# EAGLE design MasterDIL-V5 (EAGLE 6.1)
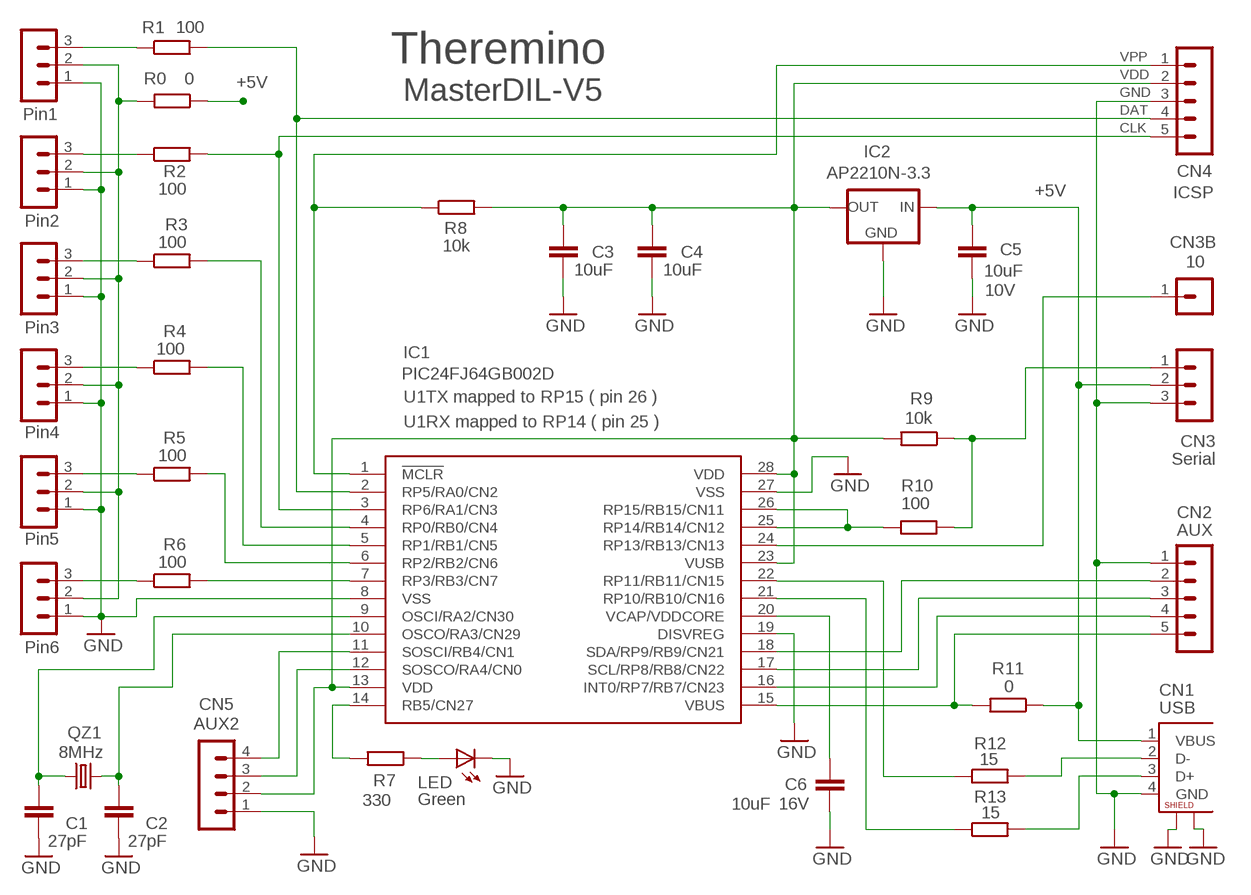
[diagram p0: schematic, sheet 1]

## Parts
C1  27pF  C-EUC0603  [C0603]
C2  27pF  C-EUC0603  [C0603]
C3  10uF  C-EUC0805  [C0805]
C4  10uF  C-EUC0805  [C0805]
C5  10uF  C-EUC0805  [C0805]
C6  10uF  C-EUC0805  [C0805]
CN1  USB  USB-BL  [USB-B-LARGE]
CN2  AUX  MA05-1  [MA05-1]
CN3  Serial  MA03-1N  [MA03-1]
CN3B  10  MA01-1  [MA01-1]
CN4  ICSP  MA05-1  [MA05-1]
CN5  AUX2  MA04-1  [MA04-1]
IC1  PIC24FJ64GB002D  [DIL28-3]
IC2  AP2210N-3.3  MCP1700SOT23L  [SOT23_L]
LED  Green  LEDLED3MM  [LED3MM]
QZ1  8MHz  CRYSTALHC49U70  [HC49U70]
R0  0  R-EU_R1206_L  [R1206_L]
R1  100  R-EU_R1206_L  [R1206_L]
R2  100  R-EU_R0805  [R0805]
R3  100  R-EU_R0805  [R0805]
R4  100  R-EU_R0805  [R0805]
R5  100  R-EU_R0805  [R0805]
R6  100  R-EU_R0805  [R0805]
R7  330  R-EU_R0805  [R0805]
R8  10k  R-EU_R0805  [R0805]
R9  10k  R-EU_R1206_L  [R1206_L]
R10  100  R-EU_R0805  [R0805]
R11  0  R-EU_R2512W  [R2512W]
R12  15  R-EU_R1206_L  [R1206_L]
R13  15  R-EU_R1206_L  [R1206_L]
SV1  Pin1  MA03-1L1  [MA03-1_L1]
SV2  Pin2  MA03-1L1  [MA03-1_L1]
SV3  Pin3  MA03-1L1  [MA03-1_L1]
SV4  Pin4  MA03-1L1  [MA03-1_L1]
SV5  Pin5  MA03-1L1  [MA03-1_L1]
SV6  Pin6  MA03-1L1  [MA03-1_L1]

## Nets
+5_PINS: R0.2 SV1.2 SV2.2 SV3.2 SV4.2 SV5.2 SV6.2
+5V: C5.1 CN1.1(VBUS) CN3.2 IC2.3(IN) R0.1 R11.1
GND: C1.2 C2.1 C3.2 C4.2 C5.2 C6.2 CN1.4(GND) CN1.G1 CN1.G2 CN2.1 CN3.3 CN4.3 CN5.1 IC1.8(VSS) IC1.19(DISVREG) IC1.27(VSS) IC2.1(GND) LED.K(C) SV1.1 SV2.1 SV3.1 SV4.1 SV5.1 SV6.1
N$1: CN4.1 IC1.1(!MCLR) R8.1
N$2: CN4.4 IC1.2(RP5/RA0/CN2) R1.2
N$3: IC1.21(RP10/RB10/CN16) R13.1
N$4: CN1.2(D-) R12.2
N$5: R1.1 SV1.3
N$6: CN4.5 IC1.3(RP6/RA1/CN3) R2.2
N$7: IC1.22(RP11/RB11/CN15) R12.1
N$8: LED.A R7.1
N$9: CN2.4 IC1.16(INT0/RP7/RB7/CN23)
N$10: CN5.3 IC1.12(SOSCO/RA4/CN0)
N$11: IC1.25(RP14/RB14/CN12) IC1.26(RP15/RB15/CN11) R10.1
N$12: CN2.3 IC1.17(SCL/RP8/RB8/CN22)
N$13: CN1.3(D+) R13.2
N$14: CN2.2 IC1.18(SDA/RP9/RB9/CN21)
N$15: CN3.1 R9.1 R10.2
N$16: C2.2 IC1.10(OSCO/RA3/CN29) QZ1.2
N$17: C1.1 IC1.9(OSCI/RA2/CN30) QZ1.1
N$18: CN3B.1 IC1.24(RP13/RB13/CN13)
N$19: IC1.7(RP3/RB3/CN7) R6.2
N$20: IC1.6(RP2/RB2/CN6) R5.2
N$21: IC1.5(RP1/RB1/CN5) R4.2
N$22: IC1.4(RP0/RB0/CN4) R3.2
N$23: R2.1 SV2.3
N$24: CN5.4 IC1.11(SOSCI/RB4/CN1)
N$25: R3.1 SV3.3
N$26: R4.1 SV4.3
N$27: R5.1 SV5.3
N$28: IC1.14(RB5/CN27) R7.2
N$29: R6.1 SV6.3
VBUS: CN2.5 IC1.15(VBUS) R11.2
VCAP/VDDCORE: C6.1 IC1.20(VCAP/VDDCORE)
VDD: C3.1 C4.1 CN4.2 CN5.2 IC1.13(VDD) IC1.23(VUSB) IC1.28(VDD) IC2.2(OUT) R8.2 R9.2

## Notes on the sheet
- Theremino
- MasterDIL-V5
- U1TX mapped to RP15 ( pin 26 )
- U1RX mapped to RP14 ( pin 25 )

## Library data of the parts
C1-C4 = 00-LIVIO:C-EU: CAPACITOR, European symbol
C5 = 00-LIVIO:C-EU: CAPACITOR, European symbol; VOLTAGE: 10V
C6 = 00-LIVIO:C-EU: CAPACITOR, European symbol; ESR: X5R; VOLTAGE: 16V
CN1 = 00-LIVIO:USB-B: USB Type-B Connector
CN2 = 03-con-lstb-M:MA05-1: PIN HEADER
CN3 SV1-SV6 = 03-con-lstb-M:MA03-1: PIN HEADER
CN3B = 03-con-lstb-M:MA01-1: PIN HEADER
CN4 = 03-con-lstb-M:MA05-1: PIN HEADER; CLK: CLK; DAT: DAT; GND: GND; VDD: VDD; VPP: VPP
CN5 = 03-con-lstb-M:MA04-1: PIN HEADER
IC1 = 00-LIVIO:PIC24FJ64GB002: PIC24FJ64GA002 edit this description Auto generated by make-symbol-device-package-bsdl.ulp Rev. 25 Source: PIC24FJ64GA002.bsd
IC2 = 00-LIVIO:MCP1700: Linear regulator Quescient courrent 1.8uA Input 2.3v to 6v Output 1.2v 1.8v 2.5v 3.0v 3.3v 5.0v
LED = 00-LIVIO:LED: LEDS
QZ1 = 00-LIVIO:CRYSTAL: CRYSTAL
R0 R1-R13 = 00-LIVIO:R-EU_: RESISTOR, European symbol

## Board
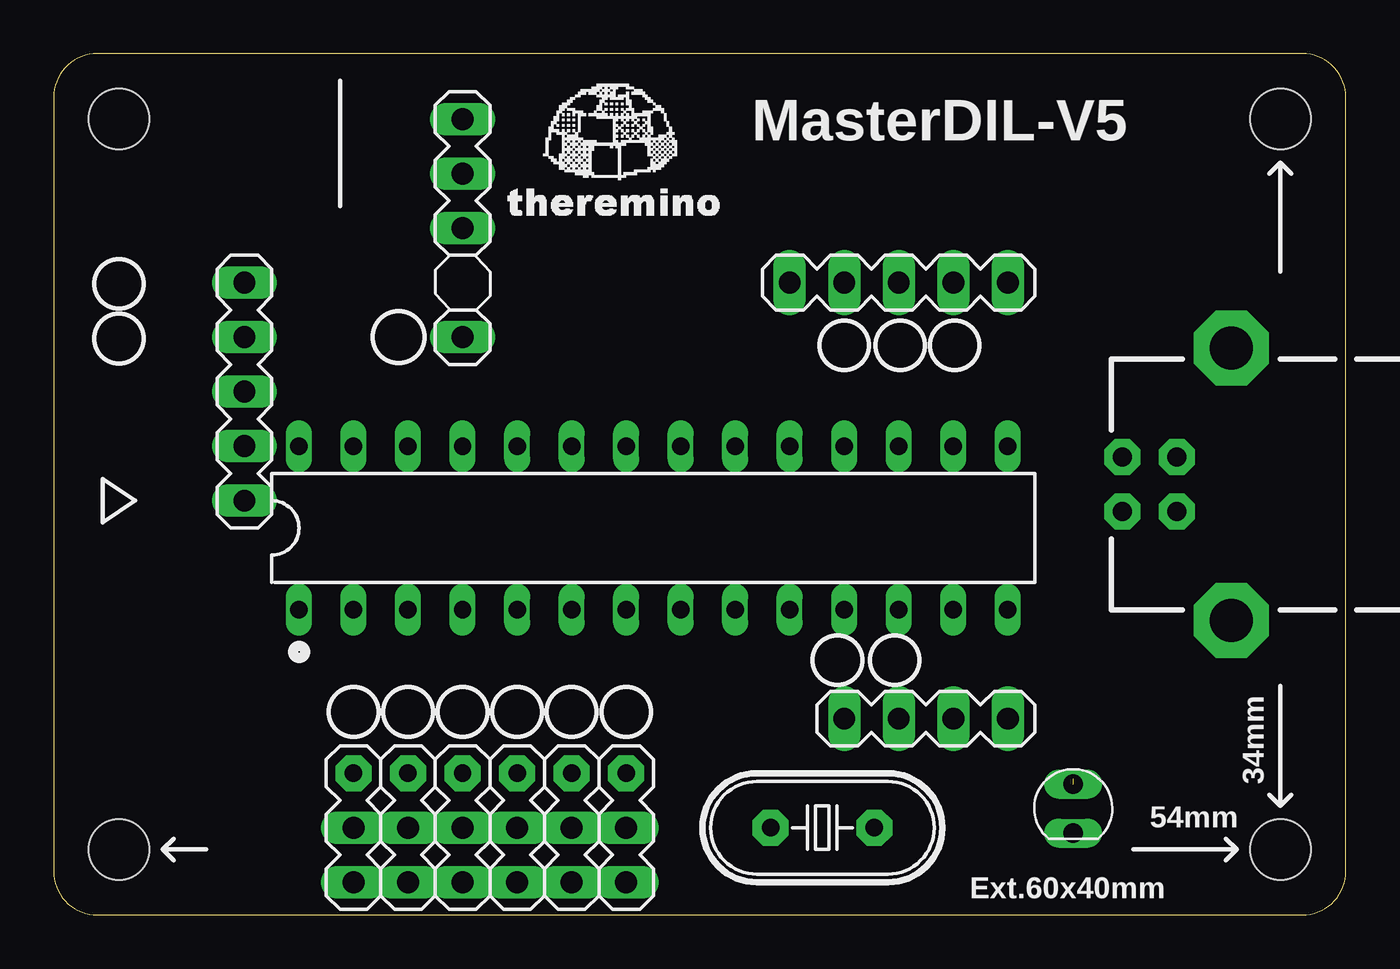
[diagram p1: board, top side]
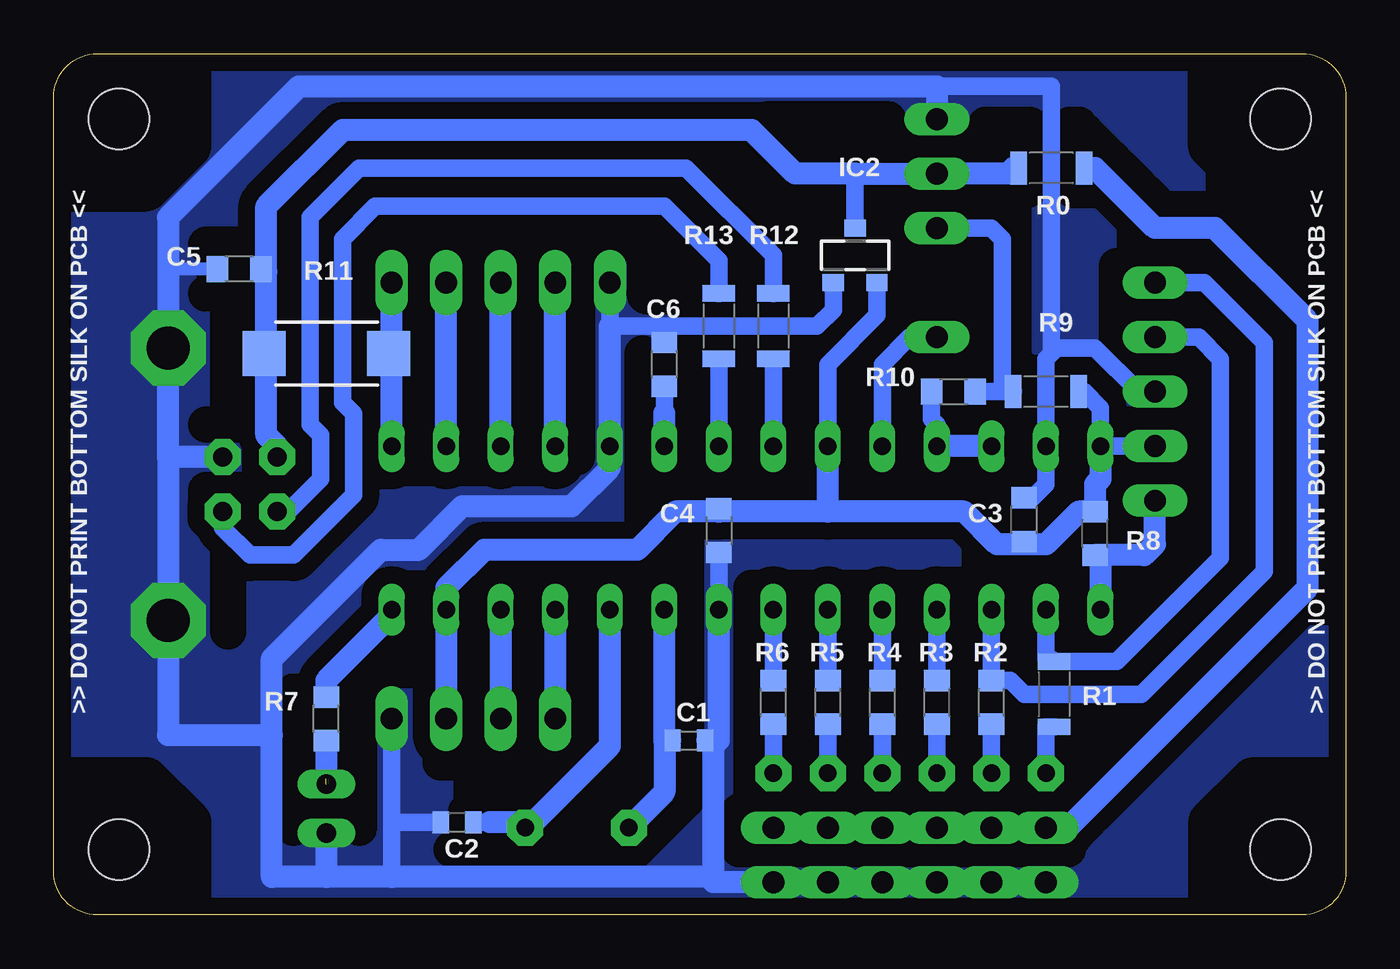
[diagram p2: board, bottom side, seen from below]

Size 60.2 x 40.13 mm. Coordinates in mm from the lower left corner, seen from the top.
Outline: 2.03,0 58.17,0 arc90 60.2,2.03 60.2,38.1 arc90 58.17,40.13 2.03,40.13 arc90 0,38.1 0,2.03 arc90 2.03,0
Copper layers (1*16): Top 0.035mm / dielectric 1.5mm / Bottom 0.035mm
Design rules: minimum track width 10mil, minimum drill 24mil, track to track 24mil, track to pad 24mil, pad to pad 24mil, via to via 24mil, smd to smd 24mil, copper to edge 24mil, drill to drill 8mil, minimum pad ring 5mil, minimum via ring 8mil, stop-mask expansion 4mil, vias tented up to drill 0mil, thermal gap 36mil
Holes 2.8 mm at 57.15,37.08 57.15,3.05 3.05,37.08 3.05,3.05
bRestrict: 67 lines

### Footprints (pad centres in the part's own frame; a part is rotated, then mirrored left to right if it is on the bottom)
C0603 = smd 0.762 x 1.016: 1 -0.762,0; 2 0.762,0
C0805 = smd 1 x 1.2: 1 -1.016,0; 2 1.016,0
USB-B-LARGE = drill 0.9 pad 1.676 octagon: 1 1.27,5.08; 2 -1.27,5.08; 3 -1.27,2.54; 4 1.27,2.54 | drill 2 pad 3.5 octagon: G1 -6.35,0; G2 6.35,0
MA05-1 = drill 1.016 long: 1 -5.08,0; 2 -2.54,0; 3 0,0; 4 2.54,0; 5 5.08,0
MA03-1 = drill 1.016 long: 1 -2.54,0; 2 0,0; 3 2.54,0
MA01-1 = drill 1.016 long: 1 0,0
MA04-1 = drill 1.016 long: 1 -3.81,0; 2 -1.27,0; 3 1.27,0; 4 3.81,0
DIL28-3 = drill 0.813 long: 1 -16.51,-3.81; 2 -13.97,-3.81; 3 -11.43,-3.81; 4 -8.89,-3.81; 5 -6.35,-3.81; 6 -3.81,-3.81; 7 -1.27,-3.81; 8 1.27,-3.81; 9 3.81,-3.81; 10 6.35,-3.81; 11 8.89,-3.81; 12 11.43,-3.81; 13 13.97,-3.81; 14 16.51,-3.81; 15 16.51,3.81; 16 13.97,3.81; 17 11.43,3.81; 18 8.89,3.81; 19 6.35,3.81; 20 3.81,3.81; 21 1.27,3.81; 22 -1.27,3.81; 23 -3.81,3.81; 24 -6.35,3.81; 25 -8.89,3.81; 26 -11.43,3.81; 27 -13.97,3.81; 28 -16.51,3.81
SOT23_L = smd 1 x 0.8: 1 -1.016,-1.27; 2 1.016,-1.27; 3 0,1.27
LED3MM = drill 0.9 long: A -1.016,0; K 1.27,0
HC49U70 = drill 0.813 pad 1.676 octagon: 1 -2.413,0; 2 2.413,0
R1206_L = smd 0.762 x 1.524: 1 -1.524,0; 2 1.524,0
R0805 = smd 1 x 1.2: 1 -1.016,0; 2 1.016,0
R2512W = smd 2 x 2.1: 1 -2.896,0; 2 2.896,0
MA03-1_L1 = drill 1.016 long: 1 -2.54,0; 2 0,0 | drill 0.813 pad 1.676 octagon: 3 2.54,0

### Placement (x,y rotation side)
C1  30.61,8.13 0 bottom
C2  41.4,4.32 0 bottom
C3  14.99,18.41 90 bottom
C4  29.21,17.91 270 bottom
C5  51.56,30.1 180 bottom
C6  31.75,25.65 90 bottom
CN1  54.86,20.07 90 top
CN2  39.37,29.46 0 top
CN3  19.05,34.54 90 top
CN3B  19.05,26.92 270 top
CN4  8.89,24.38 90 top
CN5  40.64,9.14 180 top
IC1  27.94,18.03 0 top
IC2  22.86,30.73 0 bottom
LED  47.5,5.08 270 top
QZ1  35.81,4.06 0 top
R0  13.72,34.8 0 bottom
R1  13.59,10.29 90 bottom
R2  16.51,9.91 90 bottom
R3  19.05,9.91 90 bottom
R4  21.59,9.91 90 bottom
R5  24.13,9.91 90 bottom
R6  26.67,9.91 90 bottom
R7  47.5,9.14 90 bottom
R8  11.68,17.78 90 bottom
R9  13.97,24.38 0 bottom
R10  18.29,24.38 0 bottom
R11  47.5,26.16 0 bottom
R12  26.67,27.43 90 bottom
R13  29.21,27.43 90 bottom
SV1  13.97,4.06 90 top
SV2  16.51,4.06 90 top
SV3  19.05,4.06 90 top
SV4  21.59,4.06 90 top
SV5  24.13,4.06 90 top
SV6  26.67,4.06 90 top

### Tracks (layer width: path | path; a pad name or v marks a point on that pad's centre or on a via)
+5_PINS
  Bottom 0.61: 11.94,34.8 R0.2
  Bottom 1.016: SV6.2 SV5.2 SV4.2 SV3.2 SV2.2 SV1.2 12.95,4.06 1.78,15.24 1.78,27.69 6.1,32 8.89,32 11.68,34.8 11.94,34.8
+5V
  Bottom 0.61: 15.49,34.8 R0.1 | C5.1 50.29,30.1 50.29,29.97
  Bottom 0.813: IC2.3 22.86,34.54 | R11.1 50.29,26.16
  Bottom 1.016: 15.49,34.8 15.75,34.54 CN3.2 22.86,34.54 25.65,34.54 27.69,36.58 46.74,36.58 50.29,33.02 50.29,29.97 50.29,26.16 50.29,22.35 49.78,21.84 CN1.1
GND
  Bottom 0.61: C5.2 54.86,30.1 54.86,32.51
  Bottom 0.813: 29.46,8.13 C1.2 | 34.29,27.43 31.75,27.43 | IC1.8 C4.2 | 34.29,26.16 CN2.1 | 44.45,1.78 44.45,4.32 | C2.1 44.45,4.32 | 13.46,26.42 13.97,25.91 IC1.27 13.97,20.07 14.61,19.43 C3.2 | 13.46,26.42 13.72,26.42 13.72,38.61 18.8,38.61 19.05,38.35 CN3.3 | 13.46,26.42 11.68,26.42 9.65,24.38 CN4.3 | 44.45,4.32 CN5.1 | IC2.1 23.88,28.19 24.64,27.43 31.75,27.43 | 31.75,27.43 C6.2
  Bottom 1.016: CN3.3 19.05,38.61 48.77,38.61 54.86,32.51 CN1.G2 54.86,21.34 | IC1.8 29.21,8.13 29.46,8.13 29.46,1.78 | LED.K 47.5,1.78 | 47.5,1.78 50.04,1.78 50.04,8.38 | 47.5,1.78 44.45,1.78 29.46,1.78 | 34.29,27.43 34.29,26.16 IC1.19 34.29,20.83 36.07,19.05 41.15,19.05 43.18,17.02 44.96,17.02 50.04,11.94 50.04,8.38 | SV1.1 SV2.1 SV3.1 SV4.1 SV5.1 SV6.1 29.46,1.52 29.46,1.78 | 54.86,21.34 CN1.G1 54.86,8.38 50.04,8.38 | CN1.4 54.86,21.34
  pour Bottom (isolate 0.8, no thermals): -1,-1 61.2,-1 61.2,41.13 -1,41.13
N$1
  Bottom 1.016: IC1.1 11.43,16.51 R8.1 9.4,16.76 8.89,17.27 CN4.1
N$2
  Bottom 0.813: IC1.2 13.97,11.94 13.72,11.94 R1.2 10.67,11.81 5.84,16.64 5.84,25.91 6.86,26.92 CN4.4
N$3
  Bottom 0.813: IC1.21 R13.1
N$4
  Bottom 0.813: R12.2 26.67,30.73 30.73,34.8 45.97,34.8 48.26,32.51 48.26,22.86 47.75,22.35 47.75,20.32 49.28,18.8 CN1.2
N$5
  Bottom 0.813: SV1.3 13.97,8.76 R1.1
N$6
  Bottom 0.813: CN4.5 6.6,29.46 3.81,26.67 3.81,16 9.53,10.29 14.99,10.29 15.62,10.92 R2.2 IC1.3
N$7
  Bottom 0.813: IC1.22 R12.1
N$8  (1 unrouted)
  Bottom 1.016: R7.1 47.5,6.35
N$9
  Bottom 1.016: IC1.16 CN2.4
N$10
  Bottom 1.016: IC1.12 CN5.3
N$11
  Bottom 0.813: IC1.25 19.05,22.86 19.3,23.11 R10.1
  Bottom 1.016: IC1.26 IC1.25 IC1.26
N$12
  Bottom 1.016: IC1.17 CN2.3
N$13
  Bottom 0.813: R13.2 29.21,30.48 31.75,33.02 45.21,33.02 46.74,31.5 46.74,23.88 46.23,23.37 46.23,19.56 49.02,16.76 51.05,16.76 52.32,18.03 CN1.3
N$14
  Bottom 1.016: IC1.18 CN2.2
N$15
  Bottom 0.813: 16,24.38 16,31.5 16.51,32 CN3.1 | R10.2 16,24.38 | R9.1 16,24.38
N$16
  Bottom 0.813: 39.88,4.32 C2.2
  Bottom 1.016: QZ1.2 38.1,4.06 | 39.88,4.32 38.35,4.32 38.35,4.06 QZ1.2 | QZ1.2 38.1,4.06 | 38.1,4.06 37.85,4.32 34.29,7.87 IC1.10
N$17
  Bottom 0.813: C1.1 31.75,8.13
  Bottom 1.016: QZ1.1 31.75,5.71 31.75,8.13 IC1.9
N$18
  Bottom 0.813: IC1.24 21.59,25.65 20.32,26.92 CN3B.1
N$19
  Bottom 0.813: IC1.7 R6.2
N$20
  Bottom 0.813: R5.2 24.13,13.97
  Bottom 1.016: 24.13,13.97 IC1.6
N$21
  Bottom 0.813: IC1.5 R4.2
N$22
  Bottom 0.813: IC1.4 R3.2
N$23
  Bottom 0.813: R2.1 SV2.3
N$24
  Bottom 1.016: IC1.11 CN5.4
N$25
  Bottom 0.813: R3.1 SV3.3
N$26
  Bottom 0.813: R4.1 SV4.3
N$27
  Bottom 0.813: R5.1 24.13,7.11
  Bottom 1.016: 24.13,7.11 SV5.3
N$28
  Bottom 1.016: IC1.14 44.45,13.97 47.5,10.92 R7.2
N$29
  Bottom 0.813: R6.1 SV6.3
VBUS
  Bottom 0.813: R11.2 44.45,26.16
  Bottom 1.016: IC1.15 44.45,26.16 CN2.5
VCAP/VDDCORE
  Bottom 0.813: 31.75,23.37 C6.1
  Bottom 1.016: IC1.20 31.75,23.37
VDD
  Bottom 0.61: 29.21,18.8 C4.1 | 12.19,24.38 R9.2
  Bottom 0.813: CN4.2 IC1.28 11.43,23.62 12.19,24.38 | IC1.23 24.13,25.65 21.84,27.94 IC2.2 | C3.1 14.99,17.27
  Bottom 1.016: IC1.28 11.43,20.32 11.68,20.07 R8.2 12.45,18.8 13.97,17.27 14.99,17.27 16.26,17.27 17.78,18.8 24.13,18.8 | 24.13,18.8 29.21,18.8 31.24,18.8 33.02,17.02 40.13,17.02 41.91,15.24 IC1.13 CN5.2 | 24.13,18.8 IC1.23

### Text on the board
bPlace: >> DO NOT PRINT BOTTOM SILK ON PCB << | >> DO NOT PRINT BOTTOM SILK ON PCB <<
tNames: MasterDIL-V5 | 34mm | 54mm | Ext.60x40mm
